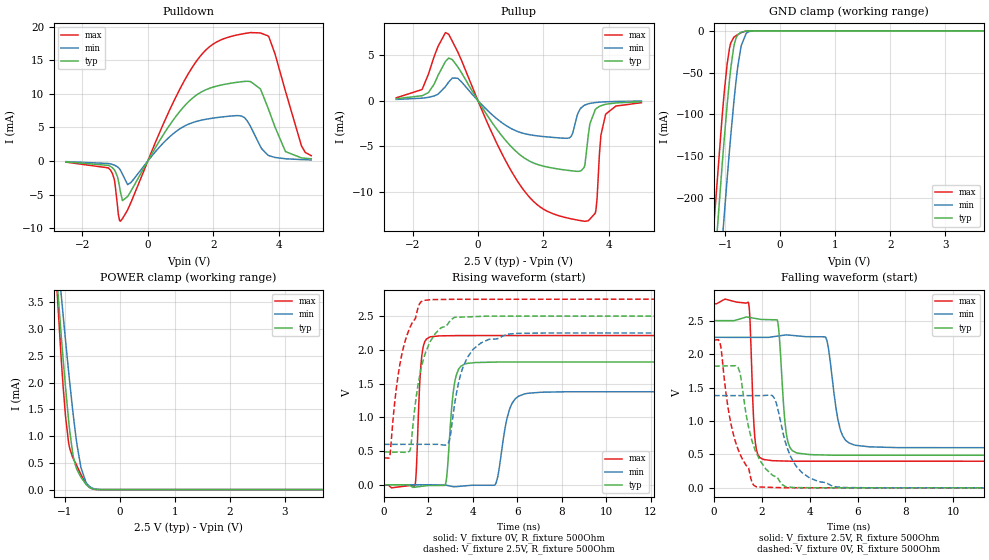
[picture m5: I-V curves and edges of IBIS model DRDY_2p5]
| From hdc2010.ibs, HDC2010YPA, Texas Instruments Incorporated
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[Model]   DRDY_2p5
Model_type   I/O
Polarity   Non-Inverting
Enable   Active-Low
Vinl = 0.75
Vinh = 1.75
Vmeas = 1.25
Vref = 2.5
Cref = 15pF
Rref = 500
|   typ   min   max
|   (nom PVT)   (slow PVT)   (fast PVT)
C_comp   0.844p   0.840p   0.852p
|C_comp (High state)   0.883p   0.878p   0.902p
|C_comp (Low state)   0.844p   0.840p   0.852p
[Model spec]
|subparameter
Vinl   0.75   0.675   0.825
Vinh   1.75   1.575   1.925
[Voltage Range]   2.5   2.25   2.75
[Temperature Range]   27   125   -40
[Pullup Reference]   2.5   2.25   2.75
[Pulldown Reference]   0   -0   0
[Power Clamp Reference]   2.5   2.25   2.75
[GND Clamp Reference]   0   0   0
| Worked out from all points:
|   slope of the pulldown table from 0 to 0.375 V, typ, clamps not added: 120 ohm
|   slope of the pullup table from 0 to 0.375 V, typ, clamps not added: 179 ohm
|   GND clamp passes 1 mA (typ) near -0.66 V on its own axis
|   POWER clamp passes 1 mA (typ) near -0.90 V on its own axis
|   falling waveform, V_fixture 2.5V, R_fixture 500Ohm: 20-80 % time 234ps typ, 392ps min, 154ps max; typ from 2.5 V to 0.487 V
|   rising waveform, V_fixture 0V, R_fixture 500Ohm: 20-80 % time 267ps typ, 436ps min, 177ps max; typ from 0 V to 1.82 V
|   rising waveform, V_fixture 2.5V, R_fixture 500Ohm: 20-80 % time 740ps typ, 754ps min, 727ps max; typ from 0.487 V to 2.5 V
|   falling waveform, V_fixture 0V, R_fixture 500Ohm: 20-80 % time 807ps typ, 841ps min, 783ps max; typ from 1.82 V to 0 V
[Pulldown]
|   Voltage   I(typ)   I(min)   I(max)
-2.5V     -130.4uA   -90.55uA   -164.7uA
-1.143V   -797.8uA   -430.8uA   -1.348mA
-1.015V   -1.364mA   -622.5uA   -3.013mA
-842.5mV  -4.491mA   -1.313mA   -8.964mA
-617.5mV  -5.293mA   -3.512mA   -7.272mA
1.445V    9.652mA    5.83mA     14.55mA
2.757V    11.73mA    6.752mA    18.77mA
3.147V    11.81mA    5.09mA     19.1mA
3.71V     7.46mA     795.5uA    18.38mA
4.213V    1.404mA    332.9uA    10.37mA
4.7V      467.6uA    212.9uA    2.272mA
5V        338uA      174.2uA    784.6uA
[GND Clamp]
|   Voltage   I(typ)   I(min)   I(max)
-2.5V     -1.538A    -1.624A    -1.483A
-1.225V   -311.8mA   -405.8mA   -251.1mA
-1.052V   -160.1mA   -252.6mA   -102mA
-1.03V    -141.4mA   -233.4mA   -84.61mA
-962.5mV  -88.72mA   -177.2mA   -39.69mA
-917.5mV  -57.63mA   -141.5mA   -20.09mA
-842.5mV  -19.45mA   -86.69mA   -7.915mA
-767.5mV  -4.696mA   -41.99mA   -4.42mA
-707.5mV  -1.712mA   -17.97mA   -2.127mA
-617.5mV  -303.7uA   -3.182mA   -305.5uA
-475mV    -7.619uA   -134.8uA   -2.409uA
5V        0A         0A         0A
[Pullup]
|   Voltage   I(typ)   I(min)   I(max)
-2.5V     209.7uA    132.6uA    307.3uA
-1.712V   534.5uA    268uA      1.212mA
-895mV    4.663mA    2.036mA    7.28mA
-617.5mV  3.705mA    2.449mA    5.341mA
1.37V     -6.163mA   -3.566mA   -9.659mA
2.795V    -7.659mA   -4.079mA   -12.91mA
3.275V    -6.991mA   -479.3uA   -13.22mA
3.425V    -2.536mA   -304.8uA   -12.99mA
3.605V    -924uA     -205.9uA   -12.08mA
3.763V    -557.6uA   -158uA     -3.787mA
3.905V    -404uA     -129.5uA   -1.521mA
5V        -121.9uA   -50.84uA   -225.4uA
[POWER Clamp]
|   Voltage   I(typ)   I(min)   I(max)
-2.5V     23.89mA    21.01mA    29.31mA
-1.24V    5.245mA    5.629mA    5.389mA
-1.067V   2.905mA    3.661mA    2.471mA
-1.06V    2.808mA    3.578mA    2.356mA
-985mV    1.884mA    2.763mA    1.345mA
-932.5mV  1.308mA    2.217mA    884.6uA
-842.5mV  597.9uA    1.355mA    571.5uA
-775mV    363.9uA    811.7uA    432.7uA
-707.5mV  230.8uA    413.3uA    282.7uA
-617.5mV  101.4uA    141.7uA    117.4uA
-520mV    23.92uA    38.7uA     21.83uA
5V        0A         0A         0A
[Ramp]
R_load = 500
|   typ   min   max
dV/dt_r   1.09128/2.66397e-10   0.827385/4.35457e-10   1.32648/1.76719e-10
dV/dt_f   1.20802/2.31458e-10   0.990622/3.88334e-10   1.41097/1.5277e-10
[Falling Waveform]
V_fixture = 2.5V
V_fixture_min = 2.25V
V_fixture_max = 2.75V
R_fixture = 500Ohm
C_fixture = 0F
|   Time   V(typ)   V(min)   V(max)
0s        2.5V       2.25V      2.749V
1.442ns   2.549V     2.249V     2.767V
1.703ns   2.534V     2.249V     757.1mV
2.023ns   2.516V     2.249V     430.5mV
2.65ns    2.499V     2.268V     404.1mV
3.011ns   836.5mV    2.286V     400.8mV
3.434ns   525.7mV    2.273V     398.7mV
4.675ns   490.7mV    2.244V     398.6mV
5.861ns   488mV      641.5mV    398.5mV
18.5ns    486.6mV    599mV      397.7mV
[Rising Waveform]
V_fixture = 0V
V_fixture_min = 0V
V_fixture_max = 0V
R_fixture = 500Ohm
C_fixture = 0F
|   Time   V(typ)   V(min)   V(max)
0s        1.01nV     30.6nV     -15.37uV
1.395ns   -34.95mV   215.5uV    -7.694mV
1.681ns   -23mV      259.7uV    1.841V
2.058ns   -10.6mV    317.9uV    2.188V
2.764ns   3.898mV    -3.844mV   2.207V
3.169ns   1.49V      -29.84mV   2.209V
3.635ns   1.788V     -16.14mV   2.21V
5.003ns   1.817V     1.61mV     2.21V
6.316ns   1.818V     1.345V     2.21V
18.5ns    1.819V     1.379V     2.211V
[Rising Waveform]
V_fixture = 2.5V
V_fixture_min = 2.25V
V_fixture_max = 2.75V
R_fixture = 500Ohm
C_fixture = 0F
|   Time   V(typ)   V(min)   V(max)
0s        486.5mV    598.9mV    397.7mV
269.2ps   484.9mV    598.9mV    433.1mV
636.6ps   482.8mV    599mV      1.621V
1.166ns   504.7mV    599.1mV    2.327V
1.442ns   1.278V     599.2mV    2.498V
1.744ns   1.818V     599.3mV    2.726V
2.854ns   2.374V     597.4mV    2.746V
3.535ns   2.484V     1.72V      2.748V
4.731ns   2.498V     2.155V     2.748V
18.5ns    2.5V       2.249V     2.75V
[Falling Waveform]
|Gnd
V_fixture = 0V
V_fixture_min = 0V
V_fixture_max = 0V
R_fixture = 500Ohm
C_fixture = 0F
|   Time   V(typ)   V(min)   V(max)
0s        1.819V     1.379V     2.211V
272.2ps   1.821V     1.379V     2.129V
636.6ps   1.824V     1.379V     1.087V
1.008ns   1.796V     1.379V     571.5mV
1.442ns   909.1mV    1.379V     297.5mV
1.762ns   524.7mV    1.379V     16.33mV
2.535ns   173.6mV    1.331V     5.812mV
3.43ns    4.349mV    325.2mV    599.9uV
5.045ns   760uV      17.88mV    543.4uV
18.5ns    86.03uV    59.07uV    72.87uV
